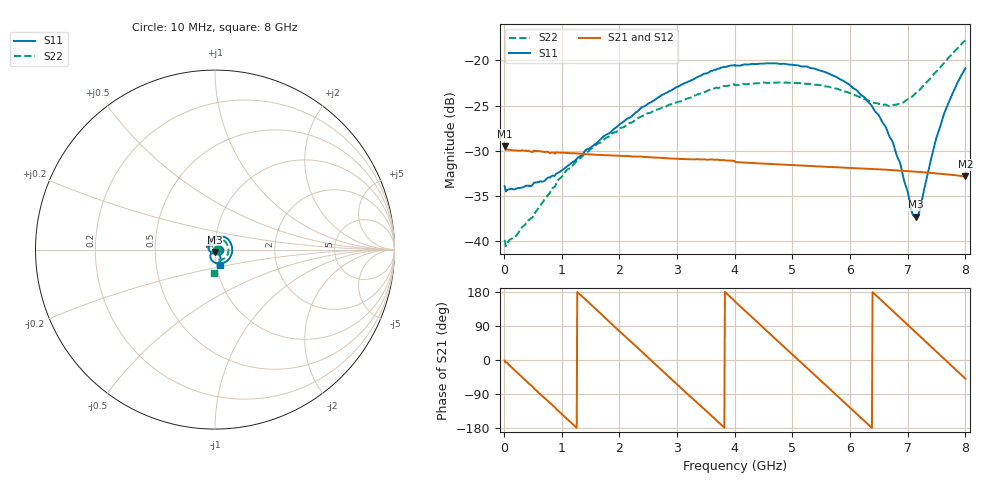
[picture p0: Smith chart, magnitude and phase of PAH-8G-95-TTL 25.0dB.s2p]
! MTS Systemtechnik GmbH
! S-Parameters
! Model: PAH-8G/95-TTL
! Attenuation Step: 25.0dB
! Rohde & Schwarz ZVB8 2Ports - Version 4.11 - 1145.1010k08 SN: 100119
! S2P File Measurements:
! S11 S21 S12 S22
# HZ  S  DB  R  50.00
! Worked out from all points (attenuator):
!   800 points, 10 MHz to 8 GHz, reference 50 ohm
!   highest |S21| = -29.49 dB at 10 MHz (marker M1); lowest = -32.8 dB at 8 GHz (marker M2)
!   lowest |S11| = -37.3 dB at 7.14 GHz (marker M3), VSWR 1.03, Z = 49.9 - j1.36 ohm
!   |S11| at or under -10 dB: start of sweep to end of sweep
!   |S22| runs from -40.6 to -17.8 dB; largest |S21 - S12| = 0.00048
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1e7  -33.91 -7.0  -29.49 -1.2  -29.40 -1.1  -39.85 -13.0
2e8  -34.22 -25.5  -29.97 -29.1  -29.97 -29.0  -39.47 -38.1
6.9e8  -33.37 -86.8  -30.12 -98.6  -30.11 -98.7  -35.50 -112.4
1.07e9  -31.84 -131.3  -30.24 -152.2  -30.24 -152.2  -32.27 -153.6
1.35e9  -30.47 -160.0  -30.34 168.3  -30.34 168.3  -30.65 -178.3
1.96e9  -27.34 151.3  -30.55 81.6  -30.56 81.8  -27.87 136.7
2.68e9  -24.07 106.8  -30.77 -19.4  -30.76 -19.1  -25.40 96.4
3.29e9  -22.08 71.7  -30.95 -104.8  -30.97 -105.2  -23.94 64.9
4.01e9  -20.60 30.1  -31.25 153.4  -31.24 153.3  -22.76 29.4
4.68e9  -20.32 -9.3  -31.48 59.2  -31.49 59.2  -22.46 -2.6
5.34e9  -20.88 -49.3  -31.70 -33.1  -31.70 -33.1  -22.64 -33.7
6.11e9  -23.28 -98.2  -31.93 -141.5  -31.95 -141.5  -23.91 -64.0
6.49e9  -26.00 -121.7  -32.05 165.0  -32.06 164.8  -24.79 -71.2
6.67e9  -28.22 -130.0  -32.11 139.5  -32.11 139.5  -25.06 -71.8
6.87e9  -31.41 -133.8  -32.19 111.1  -32.20 111.0  -24.76 -71.3
7.08e9  -36.93 -110.2  -32.29 81.3  -32.29 81.2  -23.99 -70.7
7.14e9  -37.28 -93.1  -32.32 72.7  -32.32 72.8  -23.62 -70.2
7.21e9  -36.54 -73.5  -32.35 62.8  -32.35 62.8  -23.25 -70.8
7.46e9  -29.47 -50.7  -32.48 27.4  -32.48 27.3  -21.48 -74.0
7.62e9  -26.09 -54.5  -32.57 4.7  -32.58 4.6  -20.36 -77.9
7.84e9  -22.77 -64.8  -32.72 -26.6  -32.73 -26.6  -18.81 -85.5
8e9  -20.89 -73.6  -32.84 -49.3  -32.85 -49.3  -17.80 -92.2
